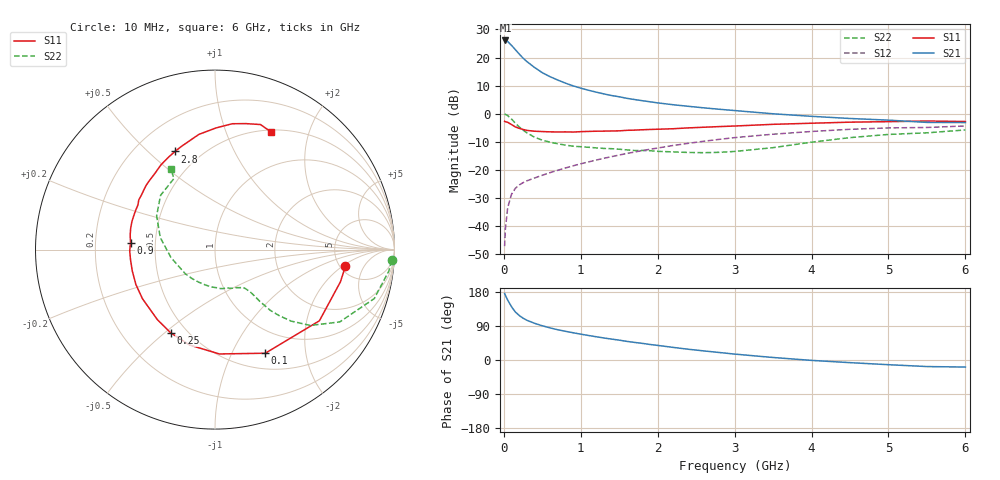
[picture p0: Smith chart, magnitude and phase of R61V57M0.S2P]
! SIEMENS Small Signal Semiconductors
! BFR193
! Si NPN RF Bipolar Junction Transistor in SOT23
! VCE = 1.5 V  IC = 7 mA
! Common Emitter S-Parameters:  May  1996
# GHz  S  MA  R  50
!  f  S11  S21  S12  S22
! GHz  MAG  ANG  MAG  ANG  MAG  ANG  MAG  ANG
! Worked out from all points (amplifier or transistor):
!   36 points, 10 MHz to 6 GHz, reference 50 ohm
!   highest |S21| = 26.1 dB at 20 MHz (marker M1)
!   |S21| within 3 dB of that: start of sweep to 140.7 MHz
!   unconditionally stable (mu >= 1): 798.3 MHz to 2.076 GHz
!   at 250 MHz: K = 0.53, MSG = 22.2 dB, |S12| = -24.5 dB
!   at 1.4 GHz: K = 1.06, MAG = 9.4 dB, |S12| = -15.3 dB
!   at 6 GHz: K = 0.97, MSG = 0.6 dB, |S12| = -4.3 dB
!   S11 on the Smith chart (normalised r, x): 10 MHz: 5.55, -2.23; 100 MHz: 0.69, -1.36; 250 MHz: 0.41, -0.52; 900 MHz: 0.36, +0.04; 2.8 GHz: 0.36, +0.61; 6 GHz: 0.52, +1.45
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0.01  0.7323 -7.3  20.05 175.7  0.0044 85.3  0.9864 -3.5
0.02  0.7216 -14.4  20.13 170.8  0.0089 82.9  0.9755 -7.1
0.05  0.704 -34.3  19.28 158.1  0.0213 73.7  0.9283 -17.1
0.1  0.6418 -64.1  16.45 140.6  0.0369 62.9  0.8033 -30.1
0.15  0.5819 -87.6  13.79 126.6  0.0472 55.7  0.6791 -38.5
0.2  0.5501 -104.9  11.55 117.5  0.054 52.4  0.5818 -43.2
0.25  0.5253 -118.1  9.759 110.3  0.0594 50.2  0.5107 -45.9
0.3  0.5052 -129.5  8.466 104.8  0.064 49.7  0.4568 -47.7
0.4  0.4881 -145.9  6.643 96.8  0.0719 50.8  0.3819 -49.1
0.5  0.4817 -156.2  5.374 90.3  0.0804 52.4  0.3384 -49.6
0.6  0.476 -165.4  4.567 84.8  0.0894 53.9  0.3123 -50.1
0.7  0.4741 -173.1  3.979 79.9  0.0985 55.3  0.2923 -51.0
0.9  0.4723 175.3  3.135 71.9  0.1183 57.5  0.2644 -53.2
1.1  0.4847 165.7  2.619 64.7  0.1387 58.5  0.2529 -57.0
1.3  0.4904 157.4  2.252 58.1  0.161 58.5  0.2414 -61.4
1.6  0.5069 146.9  1.879 49.1  0.1963 57.9  0.2272 -70.6
2.2  0.5408 128.2  1.447 33.3  0.2722 53.2  0.2094 -94.5
2.8  0.5905 112.2  1.201 19.8  0.3499 45.8  0.2057 -128.0
3.5  0.648 98.0  0.998 6.6  0.4322 34.9  0.2491 -169.7
4.5  0.7078 82.2  0.823 -7.0  0.5284 19.3  0.3758 149.9
5.5  0.7415 70.0  0.701 -17.3  0.5694 3.5  0.4573 120.0
6  0.7267 64.8  0.696 -18.6  0.6062 -1.2  0.5147 118.7
